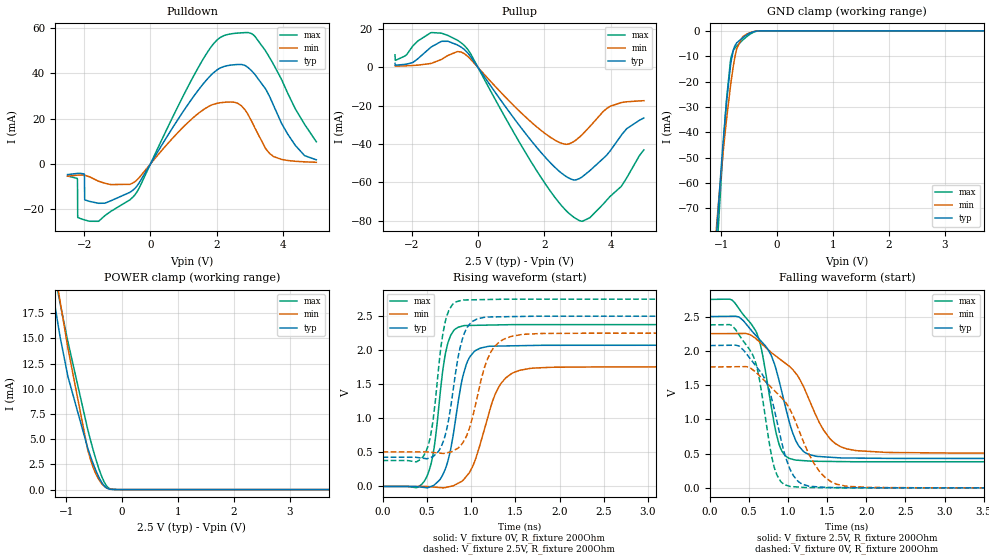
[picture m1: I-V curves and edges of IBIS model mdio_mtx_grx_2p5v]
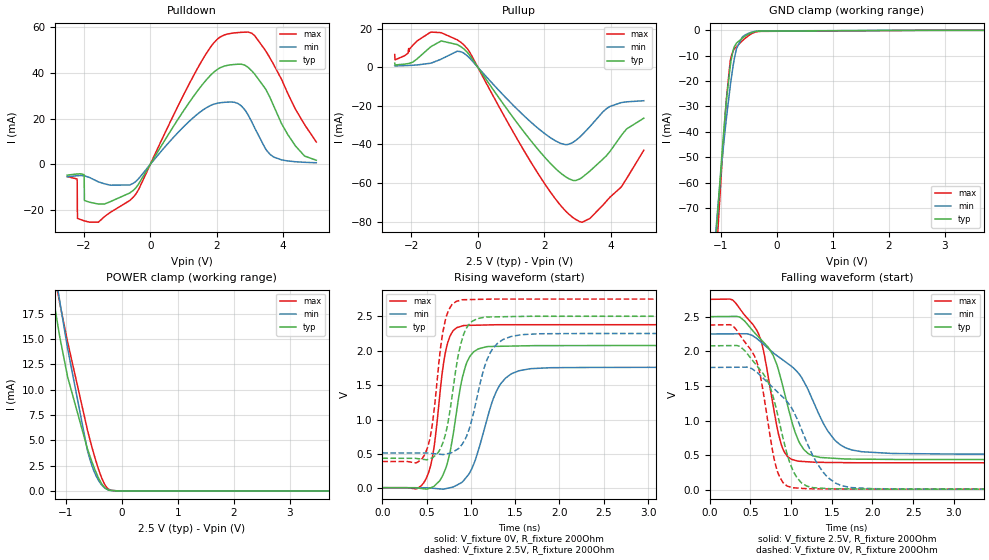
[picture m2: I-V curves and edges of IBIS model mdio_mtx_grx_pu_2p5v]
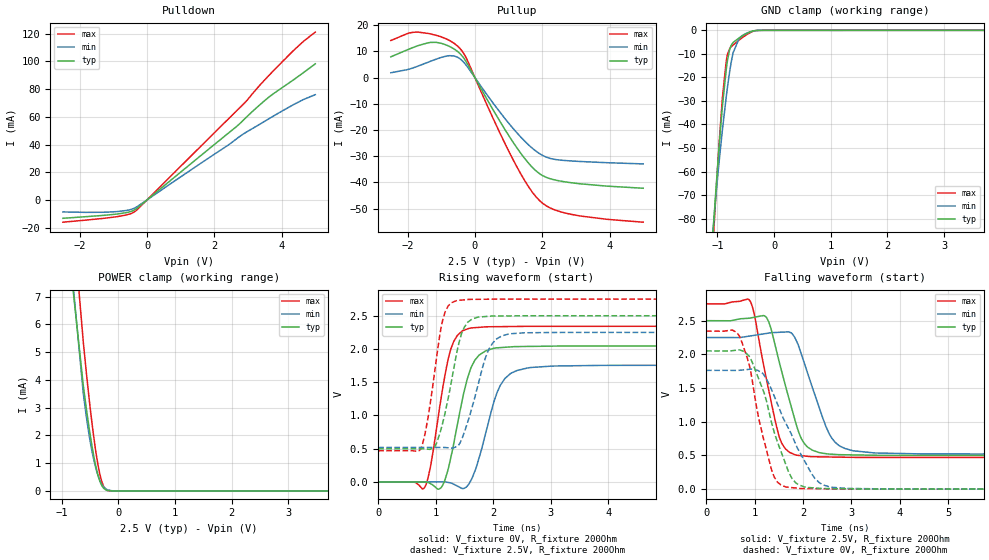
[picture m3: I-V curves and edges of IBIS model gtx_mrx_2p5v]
|Texas Instruments Incorporated
| Put part description here: 100Mbps Automotive Ethernet PHY
| Marketing Part # : DP83TC813S
| Package-type: QFN
| #pins/pkg drawing : 28-pin
[IBIS Ver] 4.1
[File name] dp83tc813_sgmii.ibs
[File Rev] 2.0
[Date] 11/02/2020
[Source]
| Texas Instruments Incorporated.
| Bengaluru, KA - 560093
[Notes] Revision History:
| Rev 1.0: 11/02/2020
| - Initial version of the model
| - Model generated from simulations in TISPICE/SPECTRE
| - C_comp although listed in numerical order of value are
| obtained from varying PVT conditions. For PVT conditions for
| each specific value refer the buffer description under
| respective [Model]. IBIS model user is responsible for using
| appropriate C_comp to simulate for Signal Integrity.
| - Warnings regarding combined Non-monotonicity of various models have been
| reviewed and considered minor and can be ignored.
|**** Modify the following if you use [Model Selector]*****************
| - Model names with a trailing _1p8v contain the model for
| 1.8V operation. Model names with a trailing _2p5v contain the model
| for 2.5V operation.Model names with a trailing _3p3v contain the model
| for 3.3V operation.
|Rev 2.0: 04/27/2021
| - Changed models for gtx_mrx_* models
| - Added slow mode models for gtx_mrx_* models
[Disclaimer]
| This model is designed as an aid for customers of Texas Instruments.
| TI and its licensors and suppliers make no warranties, either expressed
| or implied, with respect to this model, including the warranties of
| merchantability or fitness for a particular purpose. The model is
| provided solely on an "as is" basis. The entire risk as to its quality
| and performance is with the customer.
| This model is subject to change without notice. Texas Instruments
| Incorporated is not responsible for updating this model.
[Copyright]
(C) Copyright 2019 Texas Instruments Incorporated. All rights reserved.
| Component1 DP83TC813S (per package)
[Component] DP83TC813S
[Manufacturer] Texas Instruments Incorporated
[Package] |QFN 28-pin
| variable typ min max
R_pkg 0.05 0.04 0.06
L_pkg 1.0nH 0.8nH 1.2nH
C_pkg 0.2pF 0.16pF 0.24pF
| pin number (pin name) mapping to model name
[Pin] signal_name	 model_name	R_pin	L_pin	C_pin
1	TX_CLK	rgmi_mtx_grx_pd	0.119	1.74nH	0.21pF
2	TX_CTRL	rgmi_mtx_grx_pd	0.102	1.45nH	0.21pF
3	TX_D3	rgmi_mtx_grx_pd	0.086	1.19nH	0.19pF
4	TX_D2	rgmi_mtx_grx_pd	0.079	1.07nH	0.18pF
5	TX_D1	sgmii_rx_diff	0.082	1.12nH	0.19pF
6	TX_D0	sgmii_rx_diff	0.095	1.34nH	0.21pF
7	VDDIO	POWER		0.054	1.17nH	0.27pF
8	MDIO	mdio_mtx_grx	0.114	1.65nH	0.20pF
9	MDC	mdio_mtx_grx	0.121	1.79nH	0.20pF
10	INT_N	intn		0.115	1.67nH	0.22pF
11	RESET_N	mdio_mtx_grx_pu	0.114	1.66nH	0.22pF
12	XO	NC		0.121	1.77nH	0.23pF
13	XI	NC		0.133	1.99nH	0.24pF
14	LED_1	gtx_mrx		0.143	2.17nH	0.23pF
15	VSLEEP	POWER		0.128	1.91nH	0.21pF
16	WAKE	wake		0.102	1.44nH	0.20pF
17	INH	inh		0.080	1.09nH	0.18pF
18	VDDA	POWER		0.040	0.78nH	0.22pF
19	TRD_P	NC		0.085	1.16nH	0.19pF
20	TRD_M	NC		0.100	1.40nH	0.21pF
21	RX_ER	gtx_mrx_4lvlstp	0.109	1.57nH	0.22pF
22	RX_CTRL	gtx_mrx_4lvlstp	0.127	1.88nH	0.21pF
23	VDDMAC	POWER		0.069	1.64nH	0.29pF
24	RX_D3	sgmii_tx_diff	0.133	1.98nH	0.24pF
25	RX_D2	sgmii_tx_diff	0.120	1.77nH	0.23pF
26	RX_D1	gtx_mrx		0.114	1.66nH	0.22pF
27	RX_D0	gtx_mrx		0.115	1.68nH	0.22pF
28	RX_CLK	gtx_mrx		0.121	1.79nH	0.20pF
| Use Differential pin definition for differential I/Os (If Differential pin pairs are modeled)
[Diff Pin] inv_pin vdiff tdelay_typ tdelay_min tdelay_max
25 24 100mV NA NA NA
5  6 100mV NA NA NA
|***** end of component 1 definition
| Model Selectors
|***Modify the following as it applies to a speciic model with multiple ****
|*** powver supply options or driver programmability *********
[Model Selector] mdio_mtx_grx
mdio_mtx_grx_1p8v at VDDIO 1.8V operation.
mdio_mtx_grx_2p5v at VDDIO 2.5V operation.
mdio_mtx_grx_3p3v at VDDIO 3.3V operation.
[Model Selector] mdio_mtx_grx_pu
mdio_mtx_grx_pu_1p8v at VDDIO 1.8V operation.
mdio_mtx_grx_pu_2p5v at VDDIO 2.5V operation.
mdio_mtx_grx_pu_3p3v at VDDIO 3.3V operation.
[Model Selector] gtx_mrx
gtx_mrx_1p8v at VDDIO/VDDMAC 1.8V operation.
gtx_mrx_2p5v at VDDIO/VDDMAC 2.5V operation.
gtx_mrx_3p3v at VDDIO/VDDMAC 3.3V operation.
gtx_mrx_s_1p8v for slow mode at VDDIO/VDDMAC 1.8V operation.
gtx_mrx_s_2p5v for slow mode at VDDIO/VDDMAC 2.5V operation.
gtx_mrx_s_3p3v for slow mode at VDDIO/VDDMAC 3.3V operation.
[Model Selector] gtx_mrx_4lvlstp
gtx_mrx_4lvlstp_1p8v at VDDMAC 1.8V operation.
gtx_mrx_4lvlstp_2p5v at VDDMAC 2.5V operation.
gtx_mrx_4lvlstp_3p3v at VDDMAC 3.3V operation.
gtx_mrx_4lstp_s_1p8v for slow mode at VDDIO/VDDMAC 1.8V operation.
gtx_mrx_4lstp_s_2p5v for slow mode at VDDIO/VDDMAC 2.5V operation.
gtx_mrx_4lstp_s_3p3v for slow mode at VDDIO/VDDMAC 3.3V operation.
[Model Selector] gtx_mrx_sgmioff
gtx_mrx_sgmioff_1p8v at VDDMAC 1.8V operation.
gtx_mrx_sgmioff_2p5v at VDDMAC 2.5V operation.
gtx_mrx_sgmioff_3p3v at VDDMAC 3.3V operation.
gtx_sgmioff_s_1p8v for slow mode at VDDIO/VDDMAC 1.8V operation.
gtx_sgmioff_s_2p5v for slow mode at VDDIO/VDDMAC 2.5V operation.
gtx_sgmioff_s_3p3v for slow mode at VDDIO/VDDMAC 3.3V operation.
[Model Selector] rgmi_mtx_grx_pd
rgmi_mtx_grx_pd_1p8v at VDDMAC 1.8V operation.
rgmi_mtx_grx_pd_2p5v at VDDMAC 2.5V operation.
rgmi_mtx_grx_pd_3p3v at VDDMAC 3.3V operation.
[Model Selector] mtx_grx_sgmioff
mtx_grx_sgmioff_1p8v at VDDMAC 1.8V operation.
mtx_grx_sgmioff_2p5v at VDDMAC 2.5V operation.
mtx_grx_sgmioff_3p3v at VDDMAC 3.3V operation.
[Model Selector] wake
wake_3p3v at VSLEEP 3.3V
[Model Selector] inh
inh_3p3v at VSLEEP 3.3V
[Model Selector] sgmii_tx_diff
sgmii_tx at VDDA 3.3V
[Model Selector] sgmii_rx_diff
sgmii_rx at VDDA 3.3V
[Model Selector] intn
intn_1p8v at VDDIO 1.8V
intn_2p5v at VDDIO 2.5V
intn_3p3v at VDDIO 3.3V
| Models and submodels in the file (37): mdio_mtx_grx_1p8v (I/O), mdio_mtx_grx_2p5v (I/O), mdio_mtx_grx_3p3v (I/O), mdio_mtx_grx_pu_1p8v (I/O), mdio_mtx_grx_pu_2p5v (I/O), mdio_mtx_grx_pu_3p3v (I/O), gtx_mrx_1p8v (I/O), gtx_mrx_2p5v (I/O), gtx_mrx_3p3v (I/O), gtx_mrx_4lvlstp_1p8v (I/O), gtx_mrx_4lvlstp_2p5v (I/O), gtx_mrx_4lvlstp_3p3v (I/O), gtx_mrx_sgmioff_1p8v (I/O), gtx_mrx_sgmioff_2p5v (I/O), gtx_mrx_sgmioff_3p3v (I/O), gtx_mrx_s_1p8v (I/O), gtx_mrx_s_2p5v (I/O), gtx_mrx_s_3p3v (I/O), gtx_mrx_4lstp_s_1p8v (I/O), gtx_mrx_4lstp_s_2p5v (I/O), gtx_mrx_4lstp_s_3p3v (I/O), gtx_sgmioff_s_1p8v (I/O), gtx_sgmioff_s_2p5v (I/O), gtx_sgmioff_s_3p3v (I/O), rgmi_mtx_grx_pd_1p8v (I/O), rgmi_mtx_grx_pd_2p5v (I/O), rgmi_mtx_grx_pd_3p3v (I/O), mtx_grx_sgmioff_1p8v (I/O), mtx_grx_sgmioff_2p5v (I/O), mtx_grx_sgmioff_3p3v (I/O), wake_3p3v (I/O_open_source), inh_3p3v (Open_source), sgmii_rx (Input), sgmii_tx (Output), intn_1p8v (Output), intn_2p5v (Output), intn_3p3v (Output)
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| mdio_mtx_grx_2p5v
[Model]   mdio_mtx_grx_2p5v
Model_type   I/O
Polarity   Non-Inverting
Enable   Active-Low
Vinl = 0.7
Vinh = 1.7
Vmeas = 1.25
Vref = 1.25
Cref = 2pF
Rref = 100000
|   typ   min   max
C_comp   2.12pF   2.1pF   2.16pF
[Voltage Range]   2.5   2.25   2.75
[Temperature Range]   27   150   -40
[Pullup Reference]   2.5   2.25   2.75
[Pulldown Reference]   0   0   0
[Power Clamp Reference]   2.5   2.25   2.75
[GND Clamp Reference]   0   0   0
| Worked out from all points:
|   slope of the pulldown table from 0 to 0.375 V, typ, clamps not added: 41.3 ohm
|   slope of the pullup table from 0 to 0.375 V, typ, clamps not added: 39.8 ohm
|   GND clamp passes 1 mA (typ) near -0.49 V on its own axis
|   POWER clamp passes 1 mA (typ) near -0.39 V on its own axis
|   falling waveform, V_fixture 2.5V, R_fixture 200Ohm: 20-80 % time 348ps typ, 579ps min, 245ps max; typ from 2.5 V to 0.429 V
|   rising waveform, V_fixture 0V, R_fixture 200Ohm: 20-80 % time 171ps typ, 258ps min, 133ps max; typ from 0 V to 2.08 V
|   rising waveform, V_fixture 2.5V, R_fixture 200Ohm: 20-80 % time 161ps typ, 215ps min, 130ps max; typ from 0.429 V to 2.5 V
|   falling waveform, V_fixture 0V, R_fixture 200Ohm: 20-80 % time 311ps typ, 501ps min, 226ps max; typ from 2.08 V to 0 V
[Pulldown]
|   Voltage   I(typ)   I(min)   I(max)
-2.5V     -4.672mA   -5.389mA   -5.307mA
-2.208V   -4.173mA   -4.935mA   -6.345mA
-2.2V     -4.164mA   -4.928mA   -6.817mA
-2.192V   -4.156mA   -4.921mA   -23.54mA
-2.118V   -4.109mA   -4.872mA   -23.98mA
-1.99V    -4.622mA   -4.94mA    -24.62mA
-1.982V   -15.77mA   -4.953mA   -24.65mA
-617.5mV  -12.48mA   -8.98mA    -15.76mA
1.587V    35.18mA    23.8mA     46.1mA
2.428V    43.51mA    27.27mA    57.25mA
3.147V    39.41mA    15.86mA    56.18mA
5V        1.822mA    727.1uA    9.773mA
[GND Clamp]
|   Voltage   I(typ)   I(min)   I(max)
-2.5V     -599.1mA   -518.6mA   -673.8mA
-1.097V   -84.59mA   -80.54mA   -94.49mA
-1.045V   -67.62mA   -66.75mA   -74.69mA
-925mV    -32.85mA   -38.98mA   -33.1mA
-902.5mV  -27.39mA   -34.41mA   -26.49mA
-835mV    -13.92mA   -21.91mA   -11.87mA
-782.5mV  -7.515mA   -13.73mA   -7.638mA
-722.5mV  -4.731mA   -6.96mA    -5.962mA
-617.5mV  -2.758mA   -2.382mA   -3.711mA
-520mV    -1.341mA   -1.064mA   -1.898mA
-287.5mV  -11.02uA   -22.34uA   -13.28uA
5V        0A         0A         0A
[Pullup]
|   Voltage   I(typ)   I(min)   I(max)
-2.5V     2.111mA    768.5uA    6.54mA
-2.2V     1.575mA    804.7uA    5.936mA
-1.96V    2.572mA    997.9uA    11.28mA
-1.39V    10.84mA    2.186mA    18.18mA
-902.5mV  13.62mA    6.256mA    16.65mA
-467.5mV  10.11mA    7.704mA    12.3mA
2.083V    -47.91mA   -35.26mA   -62.1mA
2.638V    -56.7mA    -40.12mA   -74.4mA
3.065V    -57.97mA   -36.33mA   -79.98mA
3.973V    -43.87mA   -20.44mA   -67.55mA
4.482V    -32.02mA   -17.96mA   -57.73mA
5V        -26.43mA   -17.39mA   -43.06mA
[POWER Clamp]
|   Voltage   I(typ)   I(min)   I(max)
-2.5V     127.3mA    93.84mA    171mA
-1.232V   19.27mA    22.84mA    22.01mA
-1.225V   19.01mA    22.58mA    21.78mA
-1.113V   15.22mA    18.75mA    18.53mA
-970mV    11.21mA    14.03mA    14.66mA
-617.5mV  4.153mA    3.999mA    6.016mA
-527.5mV  2.717mA    2.349mA    4.124mA
-430mV    1.395mA    1.135mA    2.314mA
-325mV    405.8uA    361.6uA    805uA
-250mV    90.46uA    108.1uA    199.1uA
-92.5mV   742.2nA    3.182uA    929.4nA
5V        0A         0A         0A
[Ramp]
R_load = 200
|   typ   min   max
dV/dt_r   1.24591/1.68994e-10   1.05843/2.56374e-10   1.42661/1.32827e-10
dV/dt_f   1.24259/3.46294e-10   1.0458/5.79955e-10   1.42145/2.44983e-10
[Falling Waveform]
V_fixture = 2.5V
V_fixture_min = 2.25V
V_fixture_max = 2.75V
R_fixture = 200Ohm
C_fixture = 0F
|   Time   V(typ)   V(min)   V(max)
0s        2.5V       2.25V      2.75V
280.4ps   2.504V     2.252V     2.741V
580.6ps   2.23V      2.182V     2.297V
660.4ps   2.131V     2.101V     2.007V
881.2ps   1.573V     1.889V     642.1mV
1.081ns   734.9mV    1.694V     408.6mV
1.209ns   518.7mV    1.442V     396.2mV
1.53ns    447.4mV    723.7mV    385.4mV
1.877ns   434.6mV    542.5mV    381.2mV
12ns      429mV      506.9mV    380.9mV
[Rising Waveform]
V_fixture = 0V
V_fixture_min = 0V
V_fixture_max = 0V
R_fixture = 200Ohm
C_fixture = 0F
|   Time   V(typ)   V(min)   V(max)
0s        565.6nV    8.812uV    272nV
492.7ps   -18.7mV    -339.4uV   124.8mV
580.6ps   17.09mV    -9.095mV   553.3mV
675.1ps   158.4mV    -19.85mV   1.649V
731.5ps   343.9mV    -9.587mV   2.073V
920.1ps   1.675V     106mV      2.361V
1.053ns   1.998V     411.6mV    2.365V
1.315ns   2.061V     1.464V     2.372V
1.663ns   2.069V     1.732V     2.375V
12ns      2.077V     1.764V     2.378V
[Rising Waveform]
V_fixture = 2.5V
V_fixture_min = 2.25V
V_fixture_max = 2.75V
R_fixture = 200Ohm
C_fixture = 0F
|   Time   V(typ)   V(min)   V(max)
0s        429mV      506.9mV    380.9mV
481.7ps   409.8mV    506.5mV    489.2mV
563.9ps   434.9mV    499.2mV    910.6mV
654.5ps   565.6mV    487.6mV    1.996V
710ps     762.9mV    489.1mV    2.427V
900.2ps   2.153V     629.3mV    2.736V
1.012ns   2.42V      995.3mV    2.74V
1.228ns   2.488V     1.983V     2.745V
1.569ns   2.496V     2.23V      2.75V
12ns      2.5V       2.25V      2.75V
[Falling Waveform]
|Gnd
V_fixture = 0V
V_fixture_min = 0V
V_fixture_max = 0V
R_fixture = 200Ohm
C_fixture = 0F
|   Time   V(typ)   V(min)   V(max)
0s        2.077V     1.764V     2.378V
280.4ps   2.081V     1.767V     2.369V
545.3ps   1.839V     1.724V     1.94V
623.6ps   1.723V     1.646V     1.631V
815.9ps   1.174V     1.429V     322.1mV
1.021ns   277.7mV    1.146V     21.14mV
1.177ns   54.31mV    723.9mV    8.027mV
1.392ns   13.76mV    251.6mV    3.59mV
1.768ns   3.868mV    21.26mV    -7.167uV
12ns      730.2nV    9.082uV    368.5nV
| mdio_mtx_grx_pu_2p5v
[Model]   mdio_mtx_grx_pu_2p5v
Model_type   I/O
Polarity   Non-Inverting
Enable   Active-Low
Vinl = 0.7
Vinh = 1.7
Vmeas = 1.25
Vref = 1.25
Cref = 2pF
Rref = 100000
|   typ   min   max
C_comp   2.12pF   2.10pF   2.15pF
[Voltage Range]   2.5   2.25   2.75
[Temperature Range]   27   150   -40
[Pullup Reference]   2.5   2.25   2.75
[Pulldown Reference]   0   0   0
[Power Clamp Reference]   2.5   2.25   2.75
[GND Clamp Reference]   0   0   0
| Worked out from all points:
|   slope of the pulldown table from 0 to 0.375 V, typ, clamps not added: 41.3 ohm
|   slope of the pullup table from 0 to 0.375 V, typ, clamps not added: 39.8 ohm
|   GND clamp passes 1 mA (typ) near -0.46 V on its own axis
|   POWER clamp passes 1 mA (typ) near -0.39 V on its own axis
|   falling waveform, V_fixture 2.5V, R_fixture 200Ohm: 20-80 % time 349ps typ, 579ps min, 245ps max; typ from 2.5 V to 0.437 V
|   rising waveform, V_fixture 0V, R_fixture 200Ohm: 20-80 % time 170ps typ, 255ps min, 133ps max; typ from 0.009 V to 2.08 V
|   rising waveform, V_fixture 2.5V, R_fixture 200Ohm: 20-80 % time 159ps typ, 213ps min, 129ps max; typ from 0.437 V to 2.5 V
|   falling waveform, V_fixture 0V, R_fixture 200Ohm: 20-80 % time 311ps typ, 502ps min, 225ps max; typ from 2.08 V to 0.009 V
[Pulldown]
|   Voltage   I(typ)   I(min)   I(max)
-2.5V     -4.672mA   -5.389mA   -5.307mA
-2.208V   -4.173mA   -4.935mA   -6.35mA
-2.2V     -4.164mA   -4.928mA   -6.841mA
-2.192V   -4.156mA   -4.921mA   -23.54mA
-2.11V    -4.108mA   -4.87mA    -24.03mA
-1.99V    -4.622mA   -4.939mA   -24.62mA
-1.982V   -15.77mA   -4.954mA   -24.65mA
-617.5mV  -12.48mA   -8.98mA    -15.76mA
1.587V    35.18mA    23.8mA     46.1mA
2.428V    43.51mA    27.27mA    57.25mA
3.147V    39.41mA    15.86mA    56.18mA
5V        1.822mA    727.1uA    9.773mA
[GND Clamp]
|   Voltage   I(typ)   I(min)   I(max)
-2.5V     -599.5mA   -518.9mA   -674.2mA
-1.097V   -84.92mA   -80.79mA   -94.91mA
-1.045V   -67.94mA   -67mA      -75.12mA
-925mV    -33.17mA   -39.22mA   -33.53mA
-902.5mV  -27.71mA   -34.65mA   -26.92mA
-835mV    -14.24mA   -22.16mA   -12.29mA
-782.5mV  -7.835mA   -13.97mA   -8.063mA
-722.5mV  -5.051mA   -7.203mA   -6.386mA
-617.5mV  -3.076mA   -2.624mA   -4.133mA
-520mV    -1.657mA   -1.304mA   -2.318mA
-280mV    -311.1uA   -247.6uA   -414.7uA
5V        0A         0A         0A
[Pullup]
|   Voltage   I(typ)   I(min)   I(max)
-2.5V     2.111mA    768.5uA    6.54mA
-2.2V     1.575mA    804.7uA    5.937mA
-1.952V   2.636mA    1.005mA    11.43mA
-1.39V    10.84mA    2.186mA    18.18mA
-1.097V   13.59mA    4.195mA    17.83mA
-467.5mV  10.11mA    7.704mA    12.3mA
2.083V    -47.91mA   -35.26mA   -62.11mA
2.638V    -56.7mA    -40.12mA   -74.4mA
3.065V    -57.97mA   -36.33mA   -79.98mA
3.973V    -43.87mA   -20.44mA   -67.55mA
4.482V    -32.02mA   -17.96mA   -57.73mA
5V        -26.43mA   -17.39mA   -43.06mA
[POWER Clamp]
|   Voltage   I(typ)   I(min)   I(max)
-2.5V     127.3mA    93.87mA    171.1mA
-1.232V   19.32mA    22.87mA    22.07mA
-1.225V   19.06mA    22.62mA    21.83mA
-1.113V   15.27mA    18.78mA    18.58mA
-970mV    11.25mA    14.06mA    14.71mA
-617.5mV  4.191mA    4.031mA    6.059mA
-550mV    3.096mA    2.741mA    4.622mA
-460mV    1.804mA    1.481mA    2.878mA
-355mV    659.1uA    555.6uA    1.208mA
-257.5mV  133.6uA    144.6uA    267.8uA
-2.5mV    259.6nA    257.3nA    320.5nA
5V        0A         0A         0A
[Ramp]
R_load = 200
|   typ   min   max
dV/dt_r   1.24136/1.67987e-10   1.05426/2.54515e-10   1.42141/1.32191e-10
dV/dt_f   1.23787/3.46257e-10   1.04138/5.80051e-10   1.41614/2.44895e-10
[Falling Waveform]
V_fixture = 2.5V
V_fixture_min = 2.25V
V_fixture_max = 2.75V
R_fixture = 200Ohm
C_fixture = 0F
|   Time   V(typ)   V(min)   V(max)
0s        2.5V       2.25V      2.75V
281.1ps   2.504V     2.252V     2.741V
581.9ps   2.229V     2.181V     2.296V
659.9ps   2.132V     2.102V     2.011V
880.3ps   1.578V     1.891V     650mV
1.08ns    742.1mV    1.697V     415.7mV
1.221ns   515mV      1.413V     403mV
1.528ns   454.5mV    729.7mV    393.9mV
1.872ns   442.2mV    549.4mV    390mV
12ns      436.8mV    514.3mV    389.7mV
[Rising Waveform]
V_fixture = 0V
V_fixture_min = 0V
V_fixture_max = 0V
R_fixture = 200Ohm
C_fixture = 0F
|   Time   V(typ)   V(min)   V(max)
0s        9.185mV    8.948mV    10.05mV
492.8ps   -9.894mV   8.599mV    135.5mV
581.9ps   27.46mV    -396.9uV   576.7mV
674.3ps   166.6mV    -11.03mV   1.655V
724.9ps   325.9mV    -1.999mV   2.049V
919.1ps   1.681V     114.6mV    2.365V
1.037ns   1.989V     367.7mV    2.37V
1.315ns   2.063V     1.475V     2.377V
1.664ns   2.072V     1.737V     2.377V
12ns      2.078V     1.766V     2.379V
[Rising Waveform]
V_fixture = 2.5V
V_fixture_min = 2.25V
V_fixture_max = 2.75V
R_fixture = 200Ohm
C_fixture = 0F
|   Time   V(typ)   V(min)   V(max)
0s        436.8mV    514.3mV    389.7mV
481.8ps   417.4mV    513.9mV    498.5mV
564ps     442.9mV    506.4mV    923mV
655ps     574.2mV    494.7mV    2.013V
709.4ps   768.7mV    496.7mV    2.433V
899.3ps   2.155V     635.7mV    2.738V
1.013ns   2.426V     1.011V     2.743V
1.224ns   2.491V     1.983V     2.749V
1.564ns   2.498V     2.231V     2.75V
12ns      2.5V       2.25V      2.75V
[Falling Waveform]
|Gnd
V_fixture = 0V
V_fixture_min = 0V
V_fixture_max = 0V
R_fixture = 200Ohm
C_fixture = 0F
|   Time   V(typ)   V(min)   V(max)
0s        2.078V     1.766V     2.379V
279.8ps   2.083V     1.769V     2.371V
545ps     1.841V     1.726V     1.943V
625ps     1.724V     1.647V     1.626V
815.9ps   1.178V     1.431V     327.8mV
1.016ns   296.6mV    1.163V     30.02mV
1.134ns   93.94mV    853.3mV    20.33mV
1.391ns   21.8mV     259.7mV    12.94mV
1.754ns   12.73mV    30.74mV    10.06mV
12ns      9.182mV    8.934mV    10.05mV
| gtx_mrx_2p5v
[Model]   gtx_mrx_2p5v
Model_type   I/O
Polarity   Non-Inverting
Enable   Active-Low
Vinl = 0.7
Vinh = 1.7
Vmeas = 1.25
Vref = 1.25
Cref = 2pF
Rref = 100000
|   typ   min   max
C_comp   2.76pF   2.73pF   2.77pF
[Voltage Range]   2.5   2.25   2.75
[Temperature Range]   27   150   -40
[Pullup Reference]   2.5   2.25   2.75
[Pulldown Reference]   0   0   0
[Power Clamp Reference]   2.5   2.25   2.75
[GND Clamp Reference]   0   0   0
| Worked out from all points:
|   slope of the pulldown table from 0 to 0.375 V, typ, clamps not added: 49.7 ohm
|   slope of the pullup table from 0 to 0.375 V, typ, clamps not added: 43.5 ohm
|   GND clamp passes 1 mA (typ) near -0.45 V on its own axis
|   POWER clamp passes 1 mA (typ) near -0.41 V on its own axis
|   falling waveform, V_fixture 2.5V, R_fixture 200Ohm: 20-80 % time 450ps typ, 504ps min, 384ps max; typ from 2.5 V to 0.498 V
|   rising waveform, V_fixture 0V, R_fixture 200Ohm: 20-80 % time 309ps typ, 350ps min, 269ps max; typ from 0 V to 2.05 V
|   rising waveform, V_fixture 2.5V, R_fixture 200Ohm: 20-80 % time 282ps typ, 339ps min, 231ps max; typ from 0.498 V to 2.5 V
|   falling waveform, V_fixture 0V, R_fixture 200Ohm: 20-80 % time 540ps typ, 693ps min, 409ps max; typ from 2.05 V to 0 V
[Pulldown]
|   Voltage   I(typ)   I(min)   I(max)
-2.5V     -13.29mA   -8.687mA   -16.1mA
-925mV    -10.31mA   -8.492mA   -12.22mA
-512.5mV  -8.603mA   -7.139mA   -10.18mA
-347.5mV  -6.835mA   -5.631mA   -8.211mA
2.638V    52.57mA    43.69mA    63.75mA
2.885V    58.13mA    47.96mA    69.7mA
3.462V    71.02mA    56.29mA    85.76mA
3.958V    80.11mA    63.42mA    98.27mA
4.633V    91.66mA    72.28mA    114.2mA
5V        98.27mA    76.01mA    121.2mA
[GND Clamp]
|   Voltage   I(typ)   I(min)   I(max)
-2.5V     -649.6mA   -557.1mA   -724.7mA
-1.097V   -92.84mA   -90.08mA   -98.6mA
-1.03V    -68.96mA   -71.19mA   -71.1mA
-962.5mV  -46.84mA   -53.94mA   -45.4mA
-917.5mV  -33.74mA   -43.48mA   -30.33mA
-835mV    -14.88mA   -26.4mA    -11.64mA
-782.5mV  -7.979mA   -17.25mA   -7.714mA
-722.5mV  -5.135mA   -9.451mA   -6.216mA
-617.5mV  -3.252mA   -3.474mA   -4.173mA
-497.5mV  -1.53mA    -1.353mA   -2.064mA
-265mV    -14.91uA   -36.81uA   -15.25uA
5V        0A         0A         0A
[Pullup]
|   Voltage   I(typ)   I(min)   I(max)
-2.5V     7.944mA    1.866mA    14.16mA
-1.847V   11.46mA    3.685mA    17.29mA
-1.315V   13.45mA    6.279mA    16.67mA
-752.5mV  11.89mA    8.383mA    14.16mA
-460mV    9.358mA    7.341mA    11.34mA
-257.5mV  5.988mA    4.704mA    7.488mA
642.5mV   -14.55mA   -11.48mA   -18.41mA
1.272V    -27.27mA   -21.43mA   -34.67mA
1.677V    -33.87mA   -26.64mA   -43.23mA
2.007V    -37.38mA   -29.68mA   -47.93mA
2.953V    -40.27mA   -31.88mA   -52.42mA
5V        -42.22mA   -32.93mA   -55.18mA
[POWER Clamp]
|   Voltage   I(typ)   I(min)   I(max)
-2.5V     111.4mA    76.2mA     154.9mA
-1.06V    12.26mA    13.09mA    16.05mA
-617.5mV  3.803mA    3.523mA    5.367mA
-557.5mV  2.879mA    2.591mA    4.147mA
-505mV    2.141mA    1.896mA    3.157mA
-445mV    1.398mA    1.242mA    2.137mA
-392.5mV  857.5uA    791.8uA    1.369mA
-347.5mV  495.5uA    495.4uA    828.3uA
-302.5mV  241.6uA    280.7uA    419.5uA
-220mV    36.63uA    73.03uA    55.79uA
-2.5mV    0A         70.1nA     0A
5V        0A         0A         0A
[Ramp]
R_load = 200
|   typ   min   max
dV/dt_r   1.2301/3.06236e-10   1.0568/3.45474e-10   1.40676/2.68668e-10
dV/dt_f   1.20124/4.50877e-10   1.03898/5.00632e-10   1.36857/3.8458e-10
[Falling Waveform]
V_fixture = 2.5V
V_fixture_min = 2.25V
V_fixture_max = 2.75V
R_fixture = 200Ohm
C_fixture = 0F
|   Time   V(typ)   V(min)   V(max)
0s        2.5V       2.25V      2.75V
910.1ps   2.539V     2.273V     2.79V
997ps     2.551V     2.283V     2.59V
1.294ns   2.482V     2.316V     1.468V
1.564ns   1.741V     2.329V     680.1mV
1.843ns   1.008V     2.236V     508.7mV
2.082ns   634.1mV    1.754V     488.7mV
2.541ns   520.9mV    826.2mV    477.6mV
3.031ns   508.5mV    570.7mV    472mV
12ns      497.9mV    518.3mV    469mV
[Rising Waveform]
V_fixture = 0V
V_fixture_min = 0V
V_fixture_max = 0V
R_fixture = 200Ohm
C_fixture = 0F
|   Time   V(typ)   V(min)   V(max)
0s        12.17uV    93.96uV    6.783uV
810.1ps   -78.74uV   216.9uV    -78.25mV
917.4ps   -28.84mV   233.2uV    271.6mV
1.161ns   30.18mV    270.1uV    1.605V
1.314ns   580.4mV    -34.01mV   2.115V
1.582ns   1.638V     -23.02mV   2.311V
1.754ns   1.908V     364.8mV    2.325V
2.117ns   2.02V      1.443V     2.335V
2.599ns   2.038V     1.714V     2.34V
12ns      2.05V      1.761V     2.345V
[Rising Waveform]
V_fixture = 2.5V
V_fixture_min = 2.25V
V_fixture_max = 2.75V
R_fixture = 200Ohm
C_fixture = 0F
|   Time   V(typ)   V(min)   V(max)
0s        497.9mV    518.3mV    469mV
737ps     498.6mV    518.8mV    491.6mV
830.5ps   496.7mV    518.9mV    796.5mV
979.9ps   523.6mV    519mV      1.645V
1.123ns   893.4mV    519mV      2.44V
1.371ns   1.964V     538.3mV    2.729V
1.557ns   2.401V     902.4mV    2.743V
1.91ns    2.491V     1.968V     2.748V
2.273ns   2.497V     2.225V     2.749V
12ns      2.5V       2.25V      2.75V
[Falling Waveform]
|Gnd
V_fixture = 0V
V_fixture_min = 0V
V_fixture_max = 0V
R_fixture = 200Ohm
C_fixture = 0F
|   Time   V(typ)   V(min)   V(max)
0s        2.051V     1.763V     2.345V
692.4ps   2.067V     1.764V     2.265V
964.2ps   1.864V     1.78V      1.564V
1.096ns   1.618V     1.75V      1.021V
1.354ns   984.5mV    1.473V     284.1mV
1.639ns   381.8mV    988.7mV    34.27mV
1.855ns   93.17mV    661.6mV    17.1mV
2.249ns   17.47mV    157.5mV    7.406mV
2.599ns   8.136mV    28.4mV     3.826mV
12ns      12.26uV    94.05uV    6.899uV
